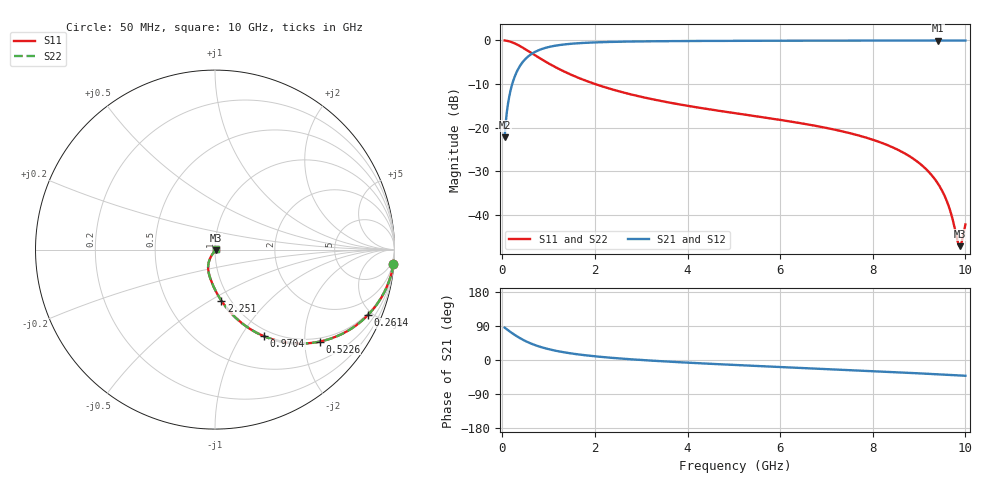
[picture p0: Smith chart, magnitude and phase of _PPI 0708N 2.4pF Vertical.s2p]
! S-Parameter data specifications (vertical orientation):
! Substrate: 40-mil Rogers 3003C, Substrate thickness, H=1.016mm, Dielectric constant, Er=3, Conductor thickness, T_mtl=0.043mm, Loss Tangent, Tand=0.003
! PCB Mounting Pad Footprint: Pad width, PadW=2.54mm , Pad length, PadL=0.51mm , Pad gap, PadG (edge-to-edge)=0.71mm , Reference planes=1.73mm apart
! Created Tue Jan 16 08:44:36 2018
# GHz S MA R 50
! 2 Port Network Data from SP1.SP block
! freq  magS11  angS11  magS21  angS21  magS12  angS12  magS22  angS22
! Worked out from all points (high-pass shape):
!   801 points, 50 MHz to 10 GHz, reference 50 ohm
!   highest |S21| = -0.04 dB at 9.415 GHz (marker M1); lowest = -22.2 dB at 50 MHz (marker M2)
!   |S21| within 3 dB of the highest: 642.1 MHz to end of sweep
!   lowest |S11| = -47.1 dB at 9.876 GHz (marker M3), VSWR 1.01, Z = 50.3 - j0.309 ohm
!   |S11| at or under -10 dB: 2.005 GHz to end of sweep
!   |S22| runs from -47.1 to 0.0 dB; largest |S21 - S12| = 0
!   S11 on the Smith chart (normalised r, x): 50 MHz: 1, -25; 261.4 MHz: 0.91, -4.69; 522.6 MHz: 0.91, -2.35; 970.4 MHz: 0.91, -1.27; 2.251 GHz: 0.91, -0.56; 10 GHz: 1.02, +0.00
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0.05  0.997 -4.7  0.07751 85.3  0.07751 85.3  0.997 -4.7
0.1495  0.974 -13.7  0.2264 76.3  0.2264 76.3  0.974 -13.7
0.2614375  0.9264 -23.2  0.3763 66.7  0.3763 66.7  0.9264 -23.2
0.373375  0.865 -31.7  0.5015 58.3  0.5015 58.3  0.865 -31.7
0.522625  0.7767 -41.3  0.6294 48.7  0.6294 48.7  0.7767 -41.3
0.7340625  0.6608 -51.8  0.75 38.2  0.75 38.2  0.6608 -51.8
0.970375  0.5559 -60.4  0.8305 29.5  0.8305 29.5  0.5559 -60.4
1.29375  0.451 -68.7  0.8917 21.2  0.8917 21.2  0.451 -68.7
1.716625  0.3597 -76.2  0.932 13.6  0.932 13.6  0.3597 -76.2
2.251438  0.287 -82.9  0.9567 6.9  0.9567 6.9  0.287 -82.9
3.370812  0.2051 -92.4  0.9772 -2.8  0.9772 -2.8  0.2051 -92.4
5.025  0.1467 -102.4  0.9872 -13.1  0.9872 -13.1  0.1467 -102.4
6.691625  0.1069 -111.0  0.9917 -22.3  0.9917 -22.3  0.1069 -111.0
7.636875  0.08315 -115.5  0.9935 -27.4  0.9935 -27.4  0.08315 -115.5
8.345812  0.06237 -118.5  0.9946 -31.4  0.9946 -31.4  0.06237 -118.5
8.980125  0.04028 -120.1  0.9953 -35.1  0.9953 -35.1  0.04028 -120.1
9.415437  0.02258 -117.8  0.9955 -37.8  0.9955 -37.8  0.02258 -117.8
9.626875  0.01324 -111.0  0.9954 -39.2  0.9954 -39.2  0.01324 -111.0
9.825875  0.005179 -73.3  0.9953 -40.5  0.9953 -40.5  0.005179 -73.3
9.875625  0.004416 -44.1  0.9952 -40.8  0.9952 -40.8  0.004416 -44.1
9.912937  0.004763 -20.3  0.9952 -41.0  0.9952 -41.0  0.004763 -20.3
10  0.007809 12.6  0.995 -41.6  0.995 -41.6  0.007809 12.6
